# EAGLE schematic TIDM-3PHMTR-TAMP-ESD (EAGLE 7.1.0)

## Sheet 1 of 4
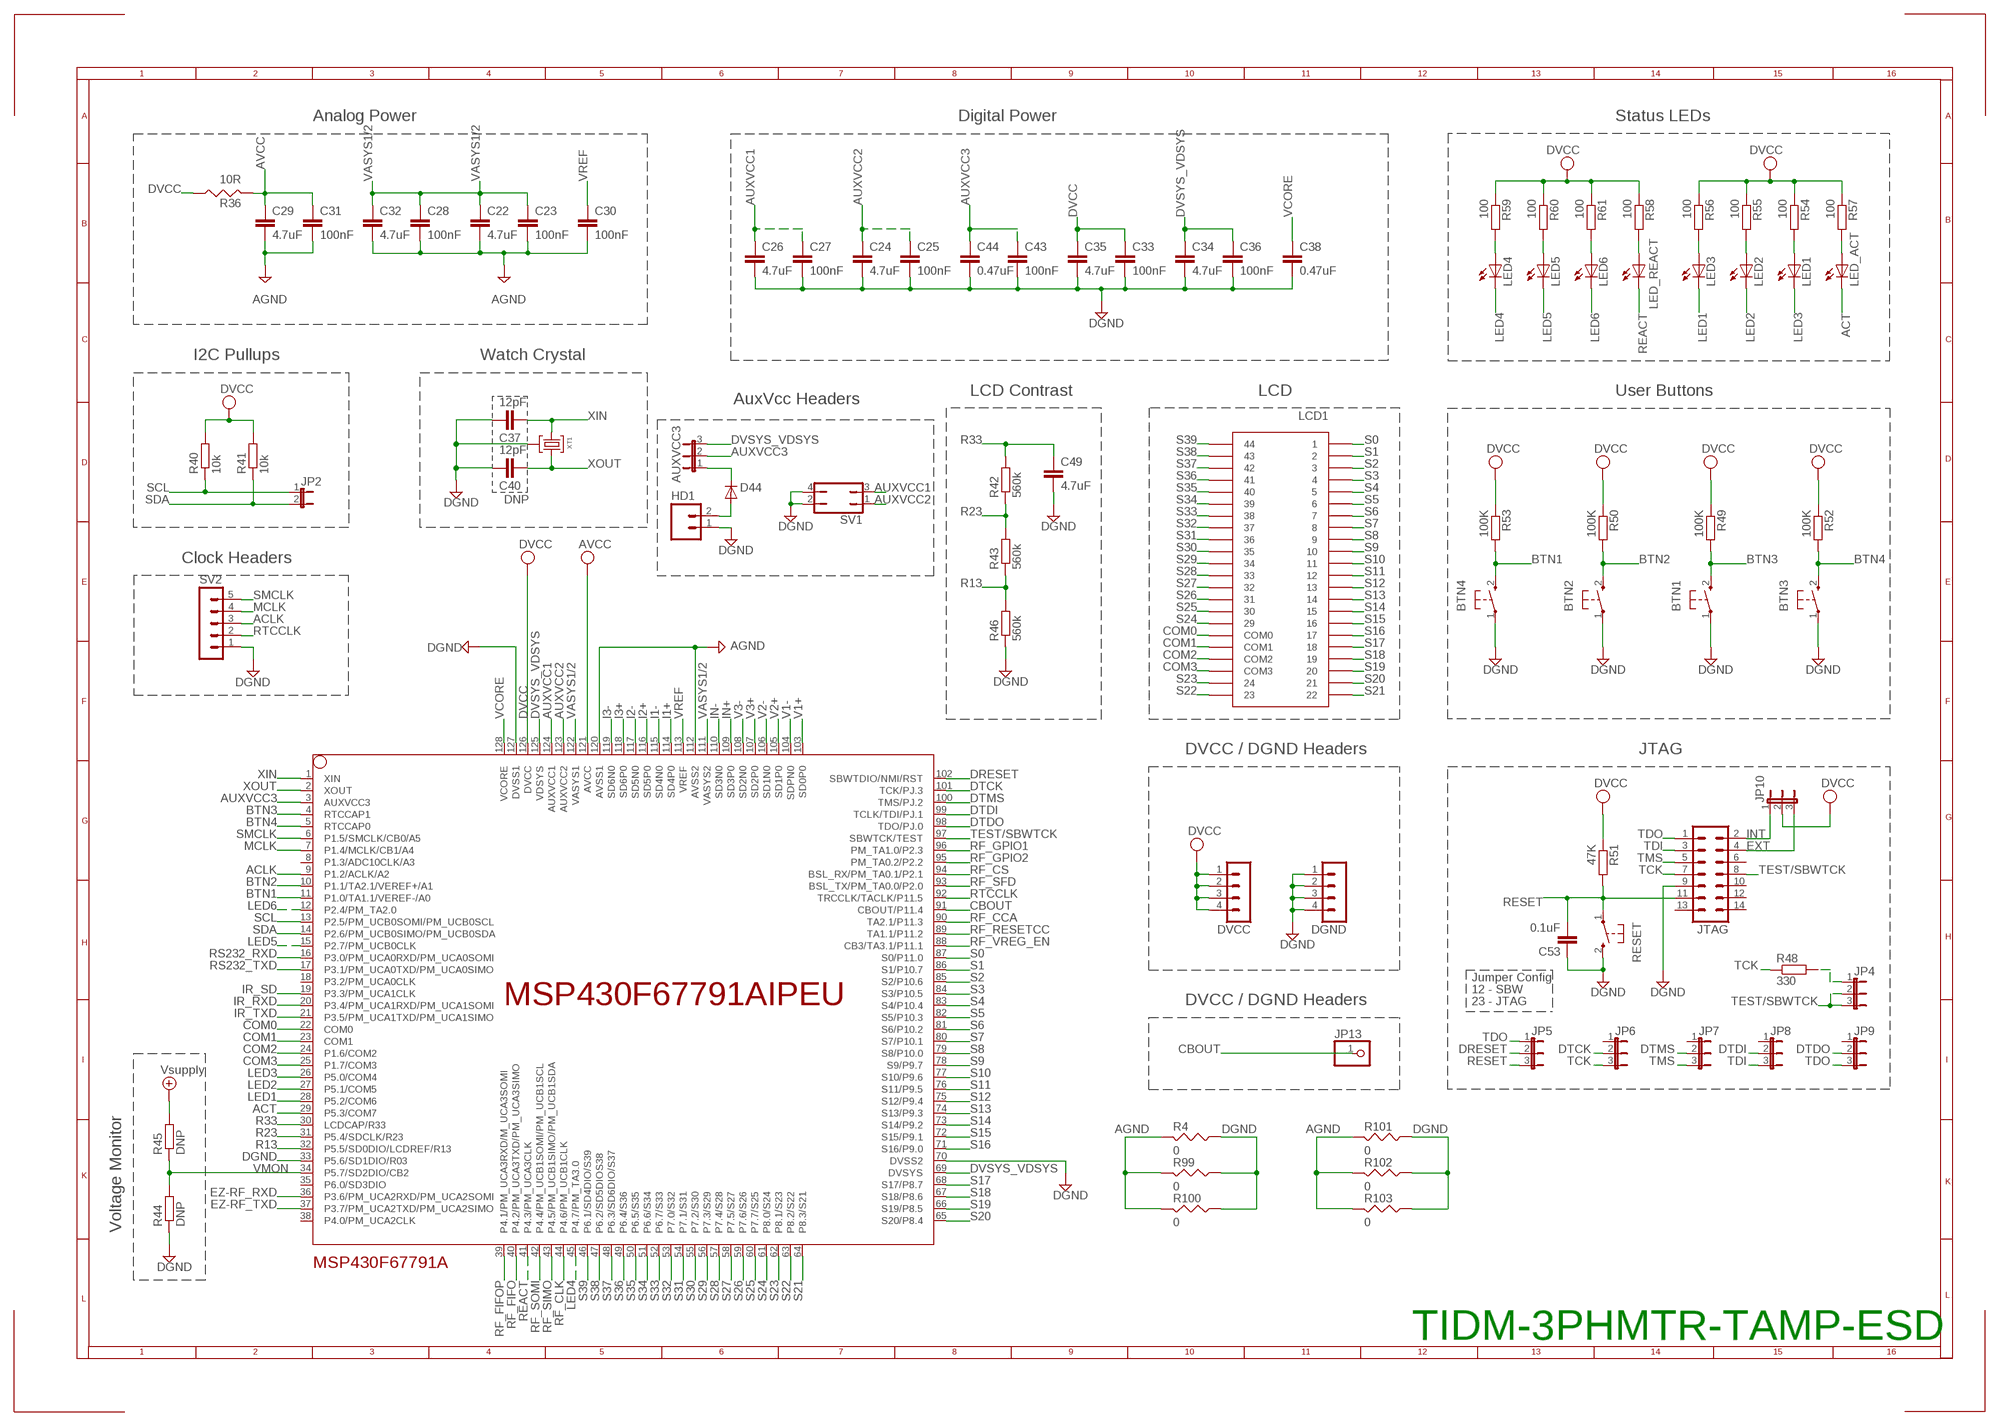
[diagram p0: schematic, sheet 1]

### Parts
AUXVCC3  JP2E  [JP2]
BTN1  PB  [PBTH]
BTN2  PB  [PBTH]
BTN3  PB  [PBTH]
BTN4  PB  [PBTH]
C22  4.7uF  C-EUC0603  [C0603]
C23  100nF  C-EUC0603  [C0603]
C24  4.7uF  C-EUC0603  [C0603]
C25  100nF  C-EUC0603  [C0603]
C26  4.7uF  C-EUC0603  [C0603]
C27  100nF  C-EUC0603  [C0603]
C28  100nF  C-EUC0603  [C0603]
C29  4.7uF  C-EUC0603  [C0603]
C30  100nF  C-EUC0603  [C0603]
C31  100nF  C-EUC0603  [C0603]
C32  4.7uF  C-EUC0603  [C0603]
C33  100nF  C-EUC0603  [C0603]
C34  4.7uF  C-EUC0603  [C0603]
C35  4.7uF  C-EUC0603  [C0603]
C36  100nF  C-EUC0603  [C0603]
C37  12pF  C-EUC0603  [C0603]
C38  0.47uF  C-EUC0603  [C0603]
C40  12pF  C-EUC0603  [C0603]
C43  100nF  C-EUC0603  [C0603]
C44  0.47uF  C-EUC0603  [C0603]
C49  4.7uF  C-EUC0603  [C0603]
C53  0.1uF  C-EUC0603  [C0603]
D44  PMLL4148  [SOD80C]
DGND  MA04-1  [MA04-1]
DVCC  MA04-1  [MA04-1]
HD1  M02PTH  [1X02]
JP2  JP1E  [JP1]
JP4  JP2E  [JP2]
JP5  JP2E  [JP2]
JP6  JP2E  [JP2]
JP7  JP2E  [JP2]
JP8  JP2E  [JP2]
JP9  JP2E  [JP2]
JP10  JP2E  [JP2]
JP13  PINHD-1X1  [1X01]
JTAG  ML14  [ML14]
LCD1  TI_160SEG_LCD  [TI_160SEG_LCD]
LED1  LED3MM  [LED3MM]
LED2  LED3MM  [LED3MM]
LED3  LED3MM  [LED3MM]
LED4  LED3MM  [LED3MM]
LED5  LED3MM  [LED3MM]
LED6  LED3MM  [LED3MM]
LED_ACT  LED3MM  [LED3MM]
LED_REACT  LED3MM  [LED3MM]
MSP430F67791A  MSP430F6779IPEU  [PEU128]
R4  0  RES0805  [R0805]
R36  10R  RES0805  [R0805]
R40  10k  R-EU_R0603  [R0603]
R41  10k  R-EU_R0603  [R0603]
R42  560k  R-EU_R0603  [R0603]
R43  560k  R-EU_R0603  [R0603]
R44  DNP  R-EU_R0603  [R0603]
R45  DNP  R-EU_R0603  [R0603]
R46  560k  R-EU_R0603  [R0603]
R48  330  R-EU_R0603  [R0603]
R49  100K  R-EU_R0603  [R0603]
R50  100K  R-EU_R0603  [R0603]
R51  47K  R-EU_R0603  [R0603]
R52  100K  R-EU_R0603  [R0603]
R53  100K  R-EU_R0603  [R0603]
R54  100  R-EU_R0603  [R0603]
R55  100  R-EU_R0603  [R0603]
R56  100  R-EU_R0603  [R0603]
R57  100  R-EU_R0603  [R0603]
R58  100  R-EU_R0603  [R0603]
R59  100  R-EU_R0603  [R0603]
R60  100  R-EU_R0603  [R0603]
R61  100  R-EU_R0603  [R0603]
R99  0  RES0805  [R0805]
R100  0  RES0805  [R0805]
R101  0  RES0805  [R0805]
R102  0  RES0805  [R0805]
R103  0  RES0805  [R0805]
RESET  PB  [PBTH]
SV1  JP2Q  [JP2Q]
SV2  MA05-1  [MA05-1]
XT1  CM200T  [CM200T]

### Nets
ACLK: MSP430F67791A.9(P1.2/ACLK/A2) SV2.3
ACT: LED_ACT.K(C) MSP430F67791A.29(P5.3/COM7) ; also sheet 4
AGND: C22.2 C23.2 C28.2 C29.2 C30.2 C31.2 C32.2 MSP430F67791A.112(AVSS2) MSP430F67791A.120(AVSS1) R4.2 R99.2 R100.2 R101.2 R102.2 R103.2 ; also sheet 2
AUXVCC1: C26.1 C27.1 MSP430F67791A.124(AUXVCC1) SV1.3
AUXVCC2: C24.1 C25.1 MSP430F67791A.123(AUXVCC2) SV1.1
AUXVCC3: AUXVCC3.2 C43.1 C44.1 MSP430F67791A.3(AUXVCC3)
AVCC: C29.1 C31.1 MSP430F67791A.121(AVCC) R36.2 ; also sheet 2
BTN1: BTN4.2(S) MSP430F67791A.11(P1.0/TA1.1/VEREF-/A0) R53.2
BTN2: BTN2.2(S) MSP430F67791A.10(P1.1/TA2.1/VEREF+/A1) R50.2
BTN3: BTN1.2(S) MSP430F67791A.4(RTCCAP1) R49.2
BTN4: BTN3.2(S) MSP430F67791A.5(RTCCAP0) R52.2
CBOUT: JP13.1 MSP430F67791A.91(CBOUT/P11.4)
COM0: LCD1.COM0 MSP430F67791A.22(COM0)
COM1: LCD1.COM1 MSP430F67791A.23(COM1)
COM2: LCD1.COM2 MSP430F67791A.24(P1.6/COM2)
COM3: LCD1.COM3 MSP430F67791A.25(P1.7/COM3)
DGND: BTN1.1(P) BTN2.1(P) BTN3.1(P) BTN4.1(P) C24.2 C25.2 C26.2 C27.2 C33.2 C34.2 C35.2 C36.2 C37.2 C38.2 C40.2 C43.2 C44.2 C49.2 C53.1 DGND.1 DGND.2 DGND.3 DGND.4 HD1.1 JTAG.9 MSP430F67791A.33(P5.6/SD1DIO/R03) MSP430F67791A.70(DVSS2) MSP430F67791A.127(DVSS1) R4.1 R44.1 R46.1 R99.1 R100.1 R101.1 R102.1 R103.1 RESET.2(S) SV1.2 SV1.4 SV2.1 XT1.P3 ; also sheet 3,4
DRESET: JP5.2 MSP430F67791A.102(SBWTDIO/NMI/RST)
DTCK: JP6.2 MSP430F67791A.101(TCK/PJ.3)
DTDI: JP8.2 MSP430F67791A.99(TCLK/TDI/PJ.1)
DTDO: JP9.2 MSP430F67791A.98(TDO/PJ.0)
DTMS: JP7.2 MSP430F67791A.100(TMS/PJ.2)
DVCC: C33.1 C35.1 DVCC.1 DVCC.2 DVCC.3 DVCC.4 JP10.2 MSP430F67791A.126(DVCC) R36.1 R40.2 R41.2 R49.1 R50.1 R51.1 R52.1 R53.1 R54.1 R55.1 R56.1 R57.1 R58.1 R59.1 R60.1 R61.1 ; also sheet 3,4
DVSYS_VDSYS: AUXVCC3.3 C34.1 C36.1 MSP430F67791A.69(DVSYS) MSP430F67791A.125(VDSYS)
EXT: JP10.3 JTAG.4
EZ-RF_RXD: MSP430F67791A.36(P3.6/PM_UCA2RXD/PM_UCA2SOMI) ; also sheet 4
EZ-RF_TXD: MSP430F67791A.37(P3.7/PM_UCA2TXD/PM_UCA2SIMO) ; also sheet 4
I1+: MSP430F67791A.114(SD4P0) ; also sheet 2
I1-: MSP430F67791A.115(SD4N0) ; also sheet 2
I2+: MSP430F67791A.116(SD5P0) ; also sheet 2
I2-: MSP430F67791A.117(SD5N0) ; also sheet 2
I3+: MSP430F67791A.118(SD6P0) ; also sheet 2
I3-: MSP430F67791A.119(SD6N0) ; also sheet 2
IN+: MSP430F67791A.109(SD3P0) ; also sheet 2
IN-: MSP430F67791A.110(SD3N0) ; also sheet 2
INT: JP10.1 JTAG.2
IR_RXD: MSP430F67791A.20(P3.4/PM_UCA1RXD/PM_UCA1SOMI) ; also sheet 4
IR_SD: MSP430F67791A.19(P3.3/PM_UCA1CLK) ; also sheet 4
IR_TXD: MSP430F67791A.21(P3.5/PM_UCA1TXD/PM_UCA1SIMO) ; also sheet 4
LED1: LED3.K(C) MSP430F67791A.28(P5.2/COM6)
LED2: LED2.K(C) MSP430F67791A.27(P5.1/COM5)
LED3: LED1.K(C) MSP430F67791A.26(P5.0/COM4)
LED4: LED4.K(C) MSP430F67791A.45(P4.7/PM_TA3.0)
LED5: LED5.K(C) MSP430F67791A.15(P2.7/PM_UCB0CLK)
LED6: LED6.K(C) MSP430F67791A.12(P2.4/PM_TA2.0)
MCLK: MSP430F67791A.7(P1.4/MCLK/CB1/A4) SV2.4
N$4: LED3.A R56.2
N$5: AUXVCC3.1 D44.C
N$7: LED2.A R55.2
N$10: JP4.1 R48.2
N$21: LED4.A R59.2
N$27: LED5.A R60.2
N$30: LED1.A R54.2
N$36: LED6.A R61.2
N$44: LED_REACT.A R58.2
N$46: LED_ACT.A R57.2
N$49: D44.A HD1.2
R13: MSP430F67791A.32(P5.5/SD0DIO/LCDREF/R13) R43.1 R46.2
R23: MSP430F67791A.31(P5.4/SDCLK/R23) R42.1 R43.2
R33: C49.1 MSP430F67791A.30(LCDCAP/R33) R42.2
REACT: LED_REACT.K(C) MSP430F67791A.41(P4.3/PM_UCA3CLK) ; also sheet 4
RESET: C53.2 JP5.3 JTAG.11 R51.2 RESET.1(P)
RF_CCA: MSP430F67791A.90(TA2.1/P11.3) ; also sheet 4
RF_CLK: MSP430F67791A.44(P4.6/PM_UCB1CLK) ; also sheet 4
RF_CS: MSP430F67791A.94(BSL_RX/PM_TA0.1/P2.1) ; also sheet 4
RF_FIFO: MSP430F67791A.40(P4.2/PM_UCA3TXD/PM_UCA3SIMO) ; also sheet 4
RF_FIFOP: MSP430F67791A.39(P4.1/PM_UCA3RXD/M_UCA3SOMI) ; also sheet 4
RF_GPIO1: MSP430F67791A.96(PM_TA1.0/P2.3) ; also sheet 4
RF_GPIO2: MSP430F67791A.95(PM_TA0.2/P2.2) ; also sheet 4
RF_RESETCC: MSP430F67791A.89(TA1.1/P11.2) ; also sheet 4
RF_SFD: MSP430F67791A.93(BSL_TX/PM_TA0.0/P2.0) ; also sheet 4
RF_SIMO: MSP430F67791A.43(P4.5/PM_UCB1SIMO/PM_UCB1SDA) ; also sheet 4
RF_SOMI: MSP430F67791A.42(P4.4/PM_UCB1SOMI/PM_UCB1SCL) ; also sheet 4
RF_VREG_EN: MSP430F67791A.88(CB3/TA3.1/P11.1) ; also sheet 4
RS232_RXD: MSP430F67791A.16(P3.0/PM_UCA0RXD/PM_UCA0SOMI) ; also sheet 4
RS232_TXD: MSP430F67791A.17(P3.1/PM_UCA0TXD/PM_UCA0SIMO) ; also sheet 4
RTCCLK: MSP430F67791A.92(TRCCLK/TACLK/P11.5) SV2.2
S0: LCD1.1 MSP430F67791A.87(S0/P11.0)
S1: LCD1.2 MSP430F67791A.86(S1/P10.7)
S2: LCD1.3 MSP430F67791A.85(S2/P10.6)
S3: LCD1.4 MSP430F67791A.84(S3/P10.5)
S4: LCD1.5 MSP430F67791A.83(S4/P10.4)
S5: LCD1.6 MSP430F67791A.82(S5/P10.3)
S6: LCD1.7 MSP430F67791A.81(S6/P10.2)
S7: LCD1.8 MSP430F67791A.80(S7/P10.1)
S8: LCD1.9 MSP430F67791A.79(S8/P10.0)
S9: LCD1.10 MSP430F67791A.78(S9/P9.7)
S10: LCD1.11 MSP430F67791A.77(S10/P9.6)
S11: LCD1.12 MSP430F67791A.76(S11/P9.5)
S12: LCD1.13 MSP430F67791A.75(S12/P9.4)
S13: LCD1.14 MSP430F67791A.74(S13/P9.3)
S14: LCD1.15 MSP430F67791A.73(S14/P9.2)
S15: LCD1.16 MSP430F67791A.72(S15/P9.1)
S16: LCD1.17 MSP430F67791A.71(S16/P9.0)
S17: LCD1.18 MSP430F67791A.68(S17/P8.7)
S18: LCD1.19 MSP430F67791A.67(S18/P8.6)
S19: LCD1.20 MSP430F67791A.66(S19/P8.5)
S20: LCD1.21 MSP430F67791A.65(S20/P8.4)
S21: LCD1.22 MSP430F67791A.64(P8.3/S21)
S22: LCD1.23 MSP430F67791A.63(P8.2/S22)
S23: LCD1.24 MSP430F67791A.62(P8.1/S23)
S24: LCD1.29 MSP430F67791A.61(P8.0/S24)
S25: LCD1.30 MSP430F67791A.60(P7.7/S25)
S26: LCD1.31 MSP430F67791A.59(P7.6/S26)
S27: LCD1.32 MSP430F67791A.58(P7.5/S27)
S28: LCD1.33 MSP430F67791A.57(P7.4/S28)
S29: LCD1.34 MSP430F67791A.56(P7.3/S29)
S30: LCD1.35 MSP430F67791A.55(P7.2/S30)
S31: LCD1.36 MSP430F67791A.54(P7.1/S31)
S32: LCD1.37 MSP430F67791A.53(P7.0/S32)
S33: LCD1.38 MSP430F67791A.52(P6.7/S33)
S34: LCD1.39 MSP430F67791A.51(P6.6/S34)
S35: LCD1.40 MSP430F67791A.50(P6.5/S35)
S36: LCD1.41 MSP430F67791A.49(P6.4/S36)
S37: LCD1.42 MSP430F67791A.48(P6.3/SD6DIO/S37)
S38: LCD1.43 MSP430F67791A.47(P6.2/SD5DIOS38)
S39: LCD1.44 MSP430F67791A.46(P6.1/SD4DIO/S39)
SCL: JP2.1 MSP430F67791A.13(P2.5/PM_UCB0SOMI/PM_UCB0SCL) R40.1 ; also sheet 4
SDA: JP2.2 MSP430F67791A.14(P2.6/PM_UCB0SIMO/PM_UCB0SDA) R41.1 ; also sheet 4
SMCLK: MSP430F67791A.6(P1.5/SMCLK/CB0/A5) SV2.5
TCK: JP6.3 JTAG.7 R48.1
TDI: JP8.3 JTAG.3
TDO: JP5.1 JP9.3 JTAG.1
TEST/SBWTCK: JP4.2 JP4.3 JTAG.8 MSP430F67791A.97(SBWTCK/TEST)
TMS: JP7.3 JTAG.5
V1+: MSP430F67791A.103(SD0P0) ; also sheet 2
V1-: MSP430F67791A.104(SDPN0) ; also sheet 2
V2+: MSP430F67791A.105(SD1P0) ; also sheet 2
V2-: MSP430F67791A.106(SD1N0) ; also sheet 2
V3+: MSP430F67791A.107(SD2P0) ; also sheet 2
V3-: MSP430F67791A.108(SD2N0) ; also sheet 2
VASYS1/2: C22.1 C23.1 C28.1 C32.1 MSP430F67791A.111(VASYS2) MSP430F67791A.122(VASYS1)
VCORE: C38.1 MSP430F67791A.128(VCORE)
VMON: MSP430F67791A.34(P5.7/SD2DIO/CB2) R44.2 R45.1
VREF: C30.1 MSP430F67791A.113(VREF)
VSUPPLY: R45.2 ; supply symbol labelled Vsupply ; also sheet 3
XIN: C37.1 MSP430F67791A.1(XIN) XT1.P2
XOUT: C40.1 MSP430F67791A.2(XOUT) XT1.P1
Unconnected: JP6.1 JP7.1 JP8.1 JP9.1 JTAG.6 JTAG.10 JTAG.12 JTAG.13 JTAG.14 MSP430F67791A.8(P1.3/ADC10CLK/A3) MSP430F67791A.18(P3.2/PM_UCA0CLK) MSP430F67791A.35(P6.0/SD3DIO) MSP430F67791A.38(P4.0/PM_UCA2CLK)

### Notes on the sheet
- Analog Power | Digital Power | Status LEDs
- I2C Pullups | Watch Crystal
- LCD Contrast | LCD | User Buttons
- AuxVcc Headers
- DNP
- Clock Headers
- DVCC / DGND Headers | JTAG
- Jumper Config
- 12 - SBW
- DVCC / DGND Headers | 23 - JTAG
- Voltage Monitor
- TIDM-3PHMTR-TAMP-ESD

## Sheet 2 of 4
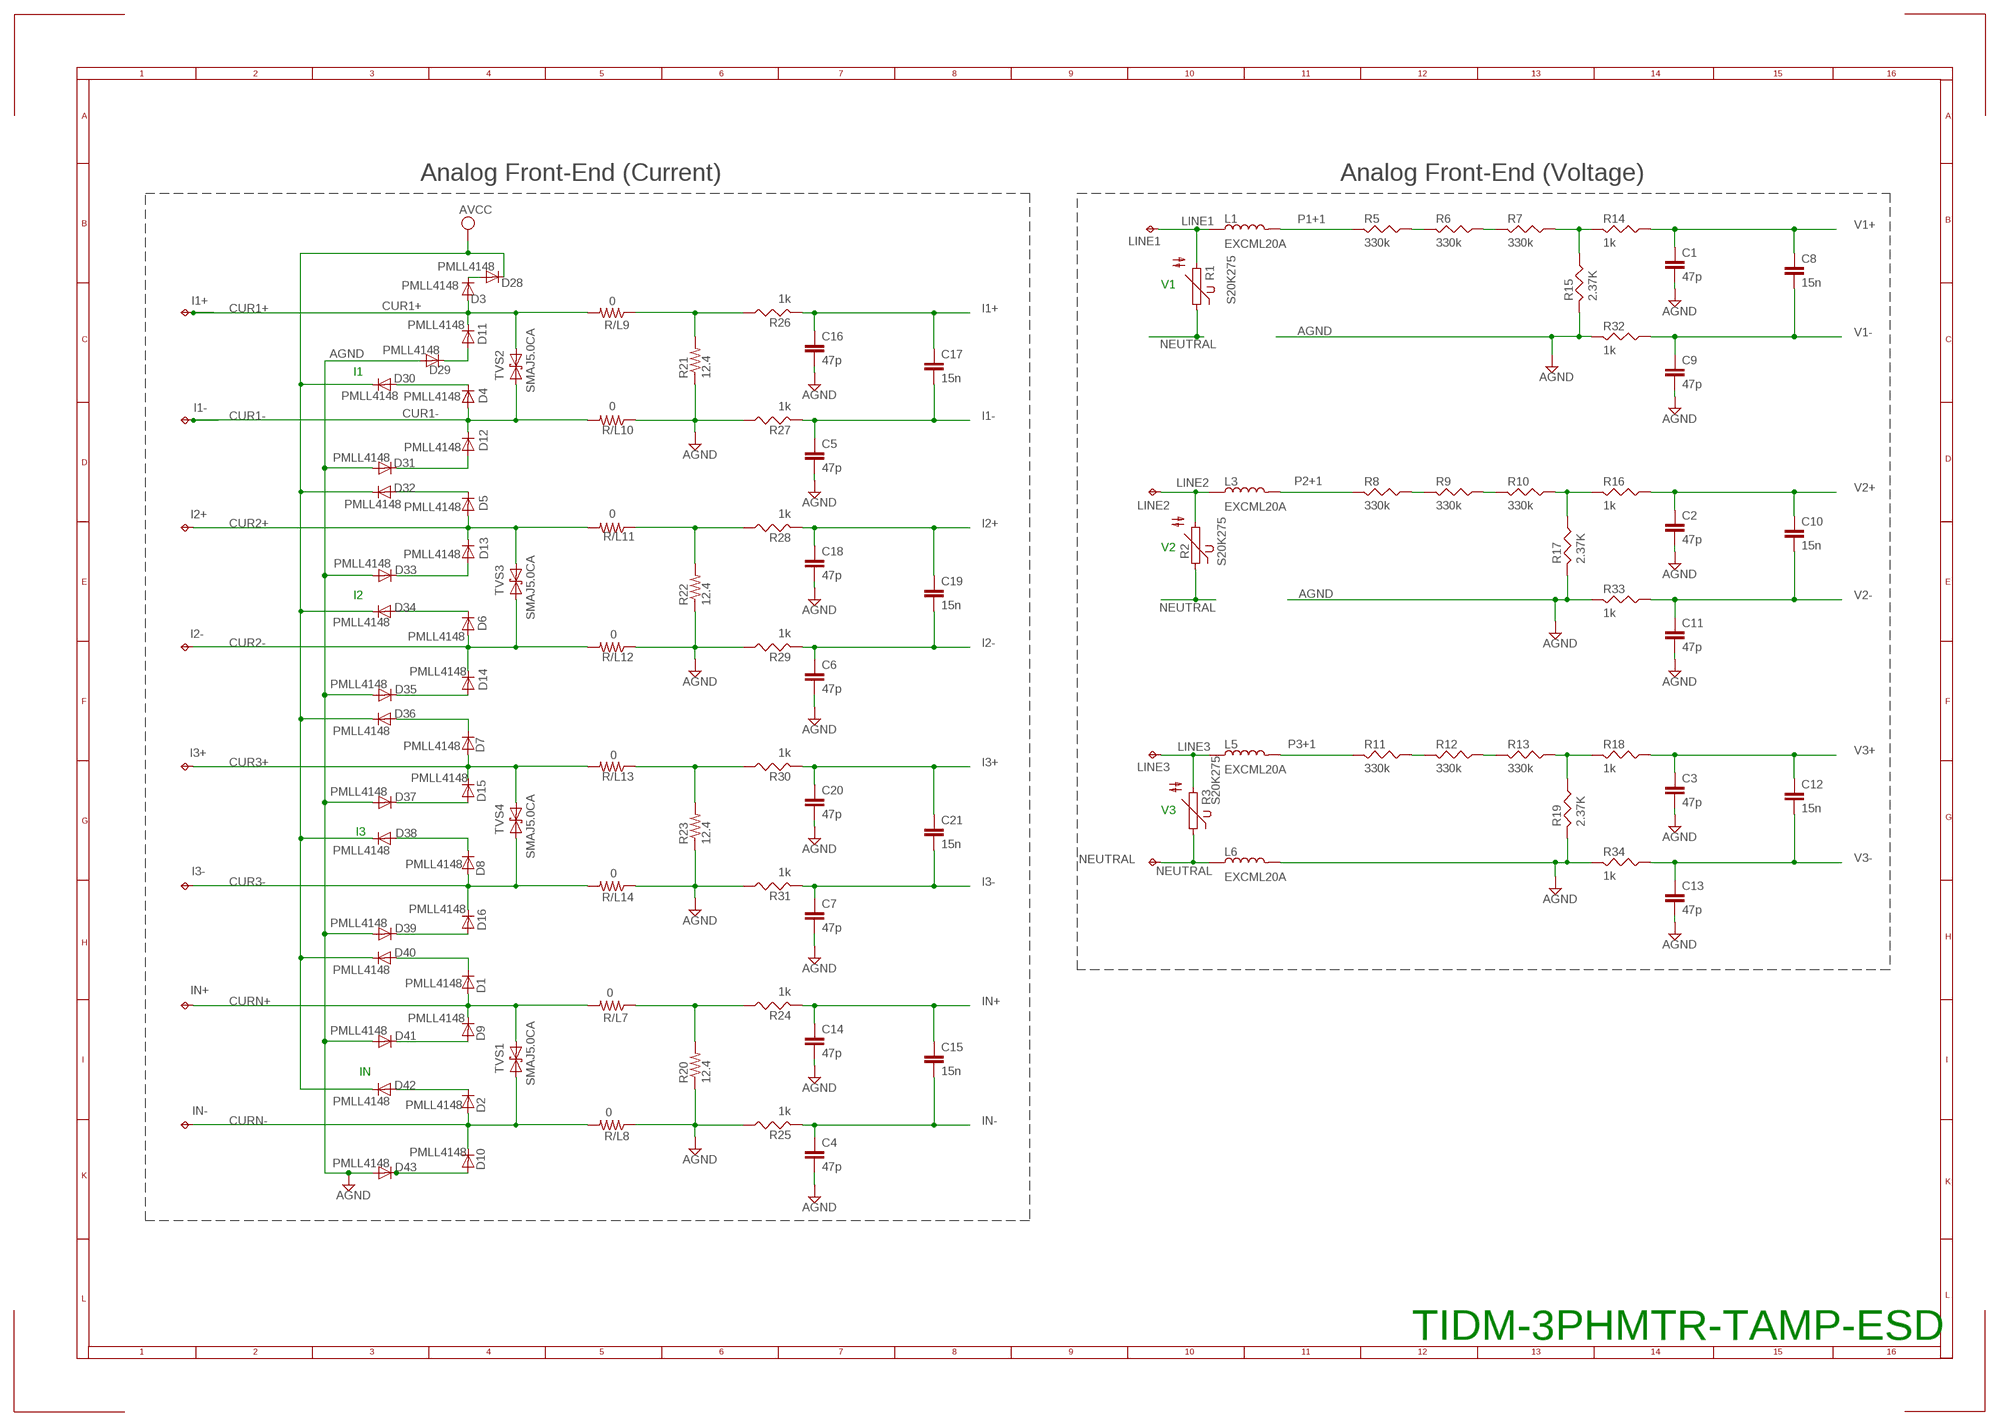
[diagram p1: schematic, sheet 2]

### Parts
C1  47p  C-EUC0805  [C0805]
C2  47p  C-EUC0805  [C0805]
C3  47p  C-EUC0805  [C0805]
C4  47p  C-EUC0805  [C0805]
C5  47p  C-EUC0805  [C0805]
C6  47p  C-EUC0805  [C0805]
C7  47p  C-EUC0805  [C0805]
C8  15n  C-EUC0805  [C0805]
C9  47p  C-EUC0805  [C0805]
C10  15n  C-EUC0805  [C0805]
C11  47p  C-EUC0805  [C0805]
C12  15n  C-EUC0805  [C0805]
C13  47p  C-EUC0805  [C0805]
C14  47p  C-EUC0805  [C0805]
C15  15n  C-EUC0805  [C0805]
C16  47p  C-EUC0805  [C0805]
C17  15n  C-EUC0805  [C0805]
C18  47p  C-EUC0805  [C0805]
C19  15n  C-EUC0805  [C0805]
C20  47p  C-EUC0805  [C0805]
C21  15n  C-EUC0805  [C0805]
D1  PMLL4148  [SOD80C]
D2  PMLL4148  [SOD80C]
D3  PMLL4148  [SOD80C]
D4  PMLL4148  [SOD80C]
D5  PMLL4148  [SOD80C]
D6  PMLL4148  [SOD80C]
D7  PMLL4148  [SOD80C]
D8  PMLL4148  [SOD80C]
D9  PMLL4148  [SOD80C]
D10  PMLL4148  [SOD80C]
D11  PMLL4148  [SOD80C]
D12  PMLL4148  [SOD80C]
D13  PMLL4148  [SOD80C]
D14  PMLL4148  [SOD80C]
D15  PMLL4148  [SOD80C]
D16  PMLL4148  [SOD80C]
D28  PMLL4148  [SOD80C]
D29  PMLL4148  [SOD80C]
D30  PMLL4148  [SOD80C]
D31  PMLL4148  [SOD80C]
D32  PMLL4148  [SOD80C]
D33  PMLL4148  [SOD80C]
D34  PMLL4148  [SOD80C]
D35  PMLL4148  [SOD80C]
D36  PMLL4148  [SOD80C]
D37  PMLL4148  [SOD80C]
D38  PMLL4148  [SOD80C]
D39  PMLL4148  [SOD80C]
D40  PMLL4148  [SOD80C]
D41  PMLL4148  [SOD80C]
D42  PMLL4148  [SOD80C]
D43  PMLL4148  [SOD80C]
I1+  TPPAD1-20  [P1-20]
I1-  TPPAD1-20  [P1-20]
I2+  TPPAD1-20  [P1-20]
I2-  TPPAD1-20  [P1-20]
I3+  TPPAD1-20  [P1-20]
I3-  TPPAD1-20  [P1-20]
IN+  TPPAD1-20  [P1-20]
IN-  TPPAD1-20  [P1-20]
L1  EXCML20A  EXCELSA390805  [R0805]
L3  EXCML20A  EXCELSA390805  [R0805]
L5  EXCML20A  EXCELSA390805  [R0805]
L6  EXCML20A  EXCELSA390805  [R0805]
LINE1  TPPAD1-20  [P1-20]
LINE2  TPPAD1-20  [P1-20]
LINE3  TPPAD1-20  [P1-20]
NEUTRAL  TPPAD1-20  [P1-20]
R1  S20K275  [S20K275]
R2  S20K275  [S20K275]
R3  S20K275  [S20K275]
R5  330k  RES0805  [R0805]
R6  330k  RES0805  [R0805]
R7  330k  RES0805  [R0805]
R8  330k  RES0805  [R0805]
R9  330k  RES0805  [R0805]
R10  330k  RES0805  [R0805]
R11  330k  RES0805  [R0805]
R12  330k  RES0805  [R0805]
R13  330k  RES0805  [R0805]
R14  1k  RES0805  [R0805]
R15  2.37K  RES0805  [R0805]
R16  1k  RES0805  [R0805]
R17  2.37K  RES0805  [R0805]
R18  1k  RES0805  [R0805]
R19  2.37K  RES0805  [R0805]
R20  12.4  R-US_R0805  [R0805]
R21  12.4  R-US_R0805  [R0805]
R22  12.4  R-US_R0805  [R0805]
R23  12.4  R-US_R0805  [R0805]
R24  1k  RES0805  [R0805]
R25  1k  RES0805  [R0805]
R26  1k  RES0805  [R0805]
R27  1k  RES0805  [R0805]
R28  1k  RES0805  [R0805]
R29  1k  RES0805  [R0805]
R30  1k  RES0805  [R0805]
R31  1k  RES0805  [R0805]
R32  1k  RES0805  [R0805]
R33  1k  RES0805  [R0805]
R34  1k  RES0805  [R0805]
R/L7  0  R-US_R0805  [R0805]
R/L8  0  R-US_R0805  [R0805]
R/L9  0  R-US_R0805  [R0805]
R/L10  0  R-US_R0805  [R0805]
R/L11  0  R-US_R0805  [R0805]
R/L12  0  R-US_R0805  [R0805]
R/L13  0  R-US_R0805  [R0805]
R/L14  0  R-US_R0805  [R0805]
TVS1  SMAJ5.0CA  [DO214AC]
TVS2  SMAJ5.0CA  [DO214AC]
TVS3  SMAJ5.0CA  [DO214AC]
TVS4  SMAJ5.0CA  [DO214AC]

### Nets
AGND: C1.2 C2.2 C3.2 C4.2 C5.2 C6.2 C7.2 C9.2 C11.2 C13.2 C14.2 C16.2 C18.2 C20.2 D29.A D31.A D33.A D35.A D37.A D39.A D41.A D43.A L6.2 R15.2 R17.2 R19.2 R20.1 R21.1 R22.1 R23.1 R25.1 R27.1 R29.1 R31.1 R32.2 R33.2 R34.2 R/L8.1 R/L10.1 R/L12.1 R/L14.1 ; also sheet 1
AVCC: D28.C D30.C D32.C D34.C D36.C D38.C D40.C D42.C ; also sheet 1
CUR1+: D3.A D11.C I1+.TP R/L9.2 TVS2.C(K)
CUR1-: D4.A D12.C I1-.TP R/L10.2 TVS2.A
CUR2+: D5.A D13.C I2+.TP R/L11.2 TVS3.C(K)
CUR2-: D6.A D14.C I2-.TP R/L12.2 TVS3.A
CUR3+: D7.A D15.C I3+.TP R/L13.2 TVS4.C(K)
CUR3-: D8.A D16.C I3-.TP R/L14.2 TVS4.A
CURN+: D1.A D9.C IN+.TP R/L7.2 TVS1.C(K)
CURN-: D2.A D10.C IN-.TP R/L8.2 TVS1.A
I1+: C16.1 C17.1 R26.2 ; also sheet 1
I1-: C5.1 C17.2 R27.2 ; also sheet 1
I2+: C18.1 C19.1 R28.2 ; also sheet 1
I2-: C6.1 C19.2 R29.2 ; also sheet 1
I3+: C20.1 C21.1 R30.2 ; also sheet 1
I3-: C7.1 C21.2 R31.2 ; also sheet 1
IN+: C14.1 C15.1 R24.2 ; also sheet 1
IN-: C4.1 C15.2 R25.2 ; also sheet 1
LINE1: L1.1 LINE1.TP R1.2
LINE2: L3.1 LINE2.TP R2.2
LINE3: L5.1 LINE3.TP R3.2
N$6: R20.2 R24.1 R/L7.1
N$8: R5.1 R6.2
N$13: R6.1 R7.2
N$14: R7.1 R14.2 R15.1
N$15: R8.1 R9.2
N$16: R9.1 R10.2
N$19: R10.1 R16.2 R17.1
N$20: D3.C D28.A
N$23: D11.A D29.C
N$25: R23.2 R30.1 R/L13.1
N$29: R11.1 R12.2
N$31: R22.2 R28.1 R/L11.1
N$32: R21.2 R26.1 R/L9.1
N$33: R12.1 R13.2
N$34: R13.1 R18.2 R19.1
N$39: D4.C D30.A
N$40: D12.A D31.C
N$42: D5.C D32.A
N$54: D13.A D33.C
N$62: D6.C D34.A
N$63: D14.A D35.C
N$64: D7.C D36.A
N$66: D15.A D37.C
N$70: D8.C D38.A
N$73: D16.A D39.C
N$74: D1.C D40.A
N$75: D9.A D41.C
N$76: D2.C D42.A
N$77: D10.A D43.C
NEUTRAL: L6.1 NEUTRAL.TP R1.1 R2.1 R3.1 ; also sheet 3
P1+1: L1.2 R5.2 ; also sheet 3
P2+1: L3.2 R8.2 ; also sheet 3
P3+1: L5.2 R11.2 ; also sheet 3
V1+: C1.1 C8.1 R14.1 ; also sheet 1
V1-: C8.2 C9.1 R32.1 ; also sheet 1
V2+: C2.1 C10.1 R16.1 ; also sheet 1
V2-: C10.2 C11.1 R33.1 ; also sheet 1
V3+: C3.1 C12.1 R18.1 ; also sheet 1
V3-: C12.2 C13.1 R34.1 ; also sheet 1

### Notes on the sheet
- Analog Front-End (Current) | Analog Front-End (Voltage)
- V1
- I1
- V2
- I2
- V3
- I3
- IN
- TIDM-3PHMTR-TAMP-ESD

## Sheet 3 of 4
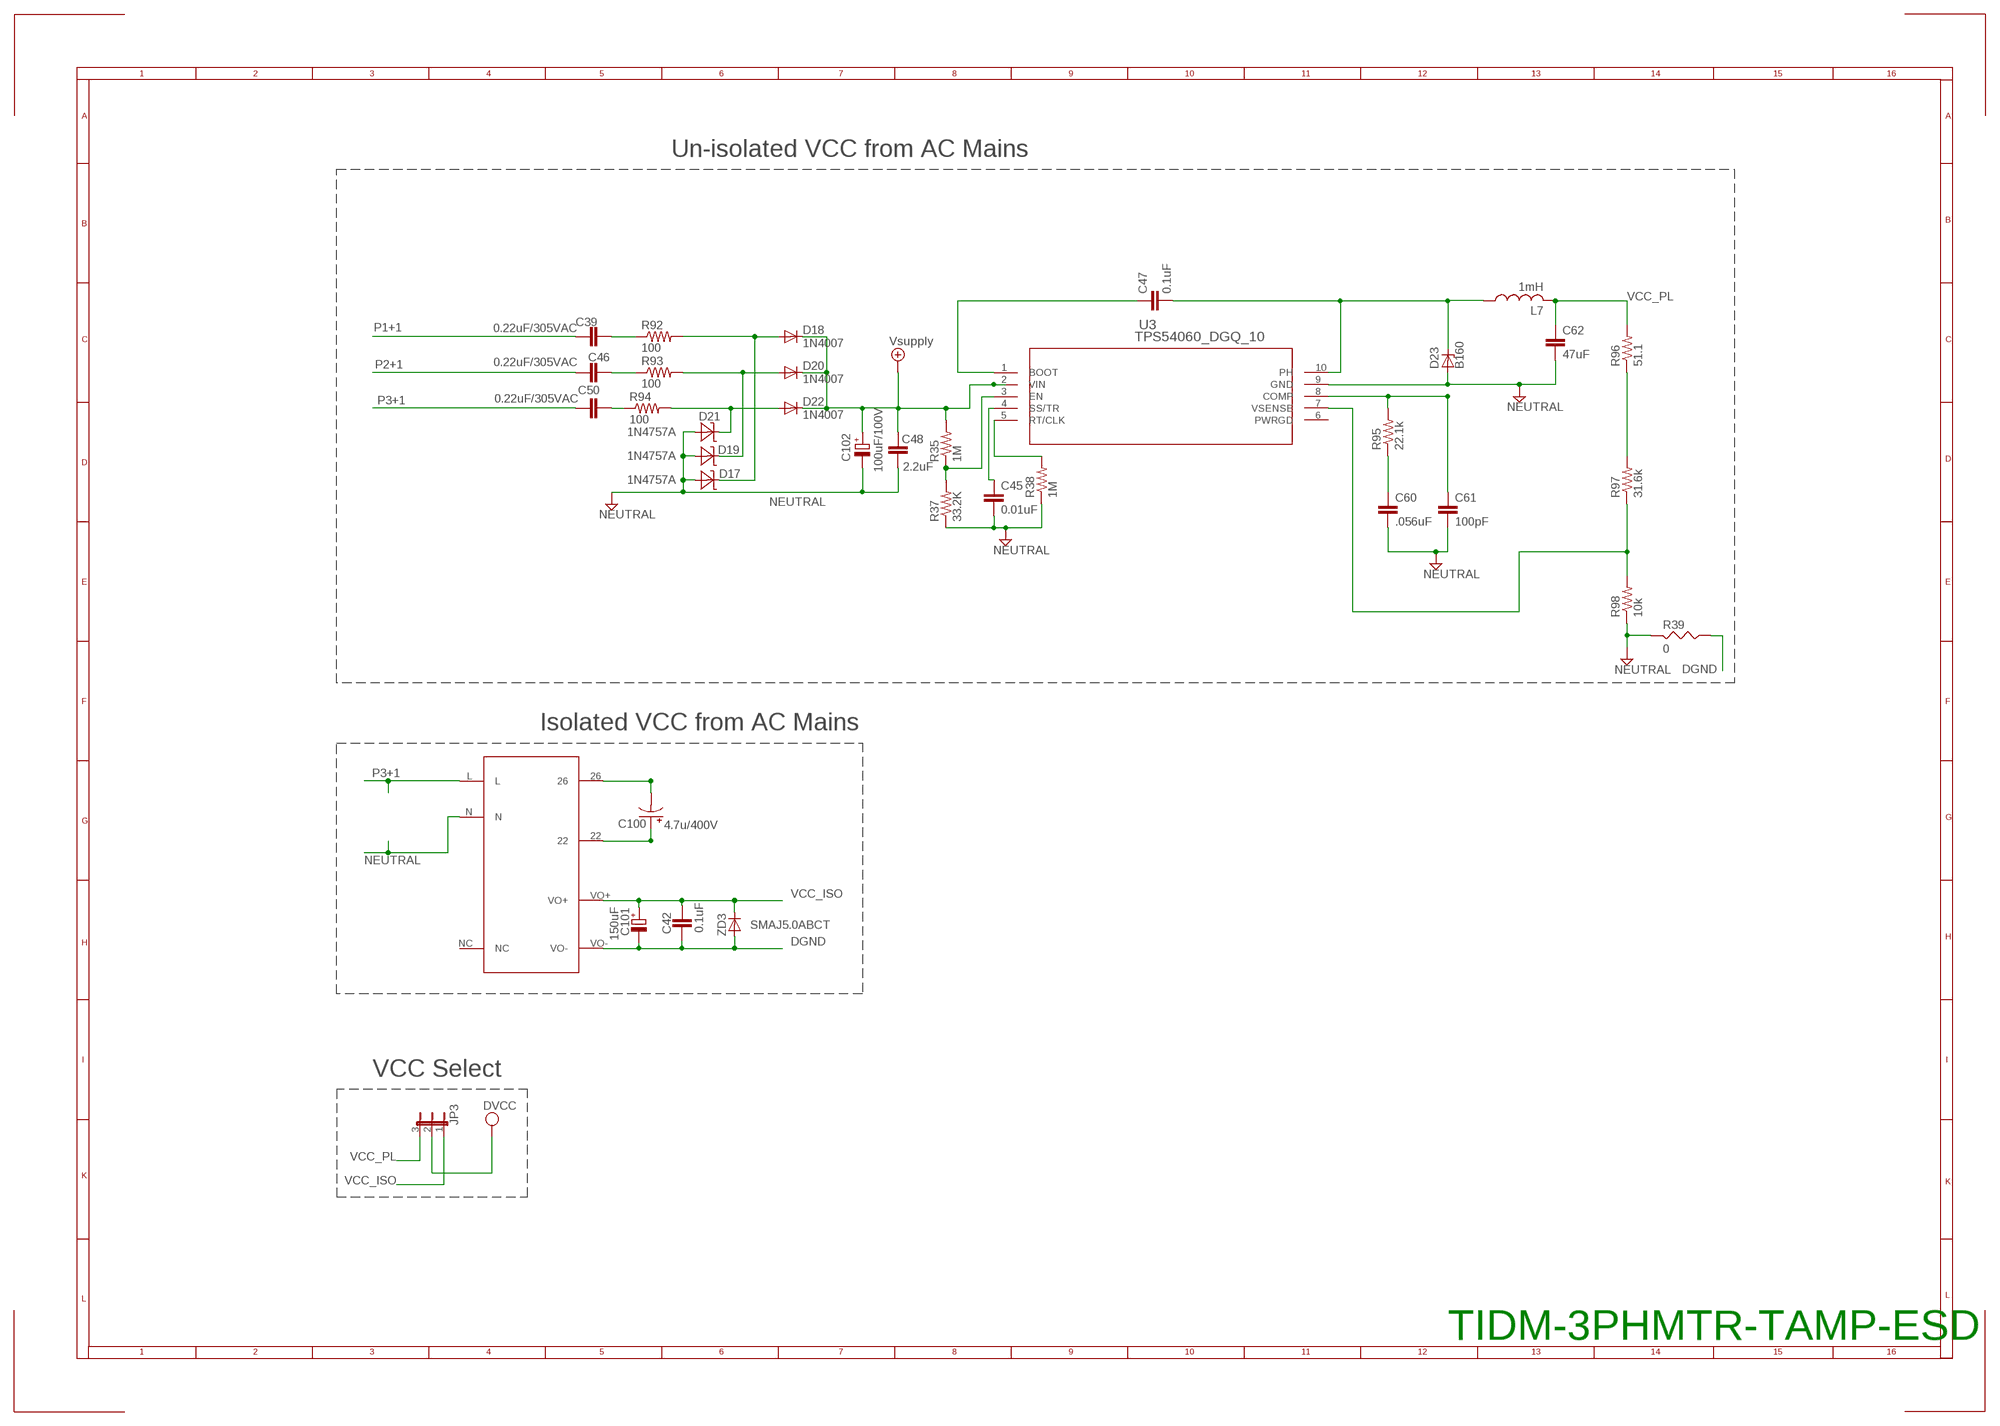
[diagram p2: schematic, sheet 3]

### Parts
C39  0.22uF/305VAC  C15/8  [C15B8]
C42  0.1uF  C-EUC0603  [C0603]
C45  0.01uF  C-EUC0603  [C0603]
C46  0.22uF/305VAC  C15/8  [C15B8]
C47  0.1uF  C-EUC0603  [C0603]
C48  2.2uF  C-EUC1210  [C1210]
C50  0.22uF/305VAC  C15/8  [C15B8]
C60  .056uF  C-EUC0603  [C0603]
C61  100pF  C-EUC0603  [C0603]
C62  47uF  C-EUC1210  [C1210]
C100  4.7u/400V  CPOL-USE5-10.5  [E5-10,5]
C101  150uF  CPOL-EUE2-5  [E2-5]
C102  100uF/100V  CPOL-EUE5-10.5  [E5-10,5]
D17  1N4757A  [DO41Z10]
D18  1N4007  [DO41-10]
D19  1N4757A  [DO41Z10]
D20  1N4007  [DO41-10]
D21  1N4757A  [DO41Z10]
D22  1N4007  [DO41-10]
D23  B160  ZENER-DIODESMB  [SMB]
JP3  JP2E  [JP2]
L7  1mH  L-USMSS1038-105  [INDUCTOR_POWER_SUPPLY_6779]
R35  1M  R-US_R0603  [R0603]
R37  33.2K  R-US_R0603  [R0603]
R38  1M  R-US_R0603  [R0603]
R39  0  RES0805  [R0805]
R92  100  R-US_0414/15  [0414/15]
R93  100  R-US_0414/15  [0414/15]
R94  100  R-US_0414/15  [0414/15]
R95  22.1k  R-US_R0603  [R0603]
R96  51.1  R-US_R0603  [R0603]
R97  31.6k  R-US_R0603  [R0603]
R98  10k  R-US_R0603  [R0603]
U3  TPS54060_DGQ_10  [DGQ10_1P88X1P57]
U$1  CUI_XR  [CUI_XR]
ZD3  SMAJ5.0ABCT  DIODE-DO214AC  [DO214AC]

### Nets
DGND: C42.2 C101.- R39.1 U$1.VO- ZD3.A ; also sheet 1,4
DVCC: JP3.2 ; also sheet 1,4
N$1: C100.- U$1.26
N$2: C100.+ U$1.22
N$17: R38.2 U3.5(RT/CLK)
N$18: D17.C D18.A R92.2
N$37: C45.1 U3.4(SS/TR)
N$38: R35.1 R37.2 U3.3(EN)
N$47: D19.C D20.A R93.2
N$78: C47.1 U3.1(BOOT)
N$80: C47.2 D23.C L7.1 U3.10(PH)
N$82: C60.1 R95.1
N$84: C39.2 R92.1
N$89: C46.2 R93.1
N$90: C50.2 R94.1
N$92: C61.1 R95.2 U3.8(COMP)
N$93: R96.1 R97.2
N$94: D21.C D22.A R94.2
N$95: R97.1 R98.2 U3.7(VSENSE)
NEUTRAL: C45.2 C48.2 C60.2 C61.2 C62.2 C102.- D17.A D19.A D21.A D23.A R37.1 R38.1 R39.2 R98.1 U3.9(GND) U$1.N ; also sheet 2
P1+1: C39.1 ; also sheet 2
P2+1: C46.1 ; also sheet 2
P3+1: C50.1 U$1.L ; also sheet 2
VCC_ISO: C42.1 C101.+ JP3.1 U$1.VO+ ZD3.C
VCC_PL: C62.1 JP3.3 L7.2 R96.2
VSUPPLY: C48.1 C102.+ D18.C D20.C D22.C R35.2 U3.2(VIN) ; supply symbol labelled Vsupply ; also sheet 1
Unconnected: U3.6(PWRGD) U$1.NC

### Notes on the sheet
- Un-isolated VCC from AC Mains
- Isolated VCC from AC Mains
- VCC Select
- TIDM-3PHMTR-TAMP-ESD

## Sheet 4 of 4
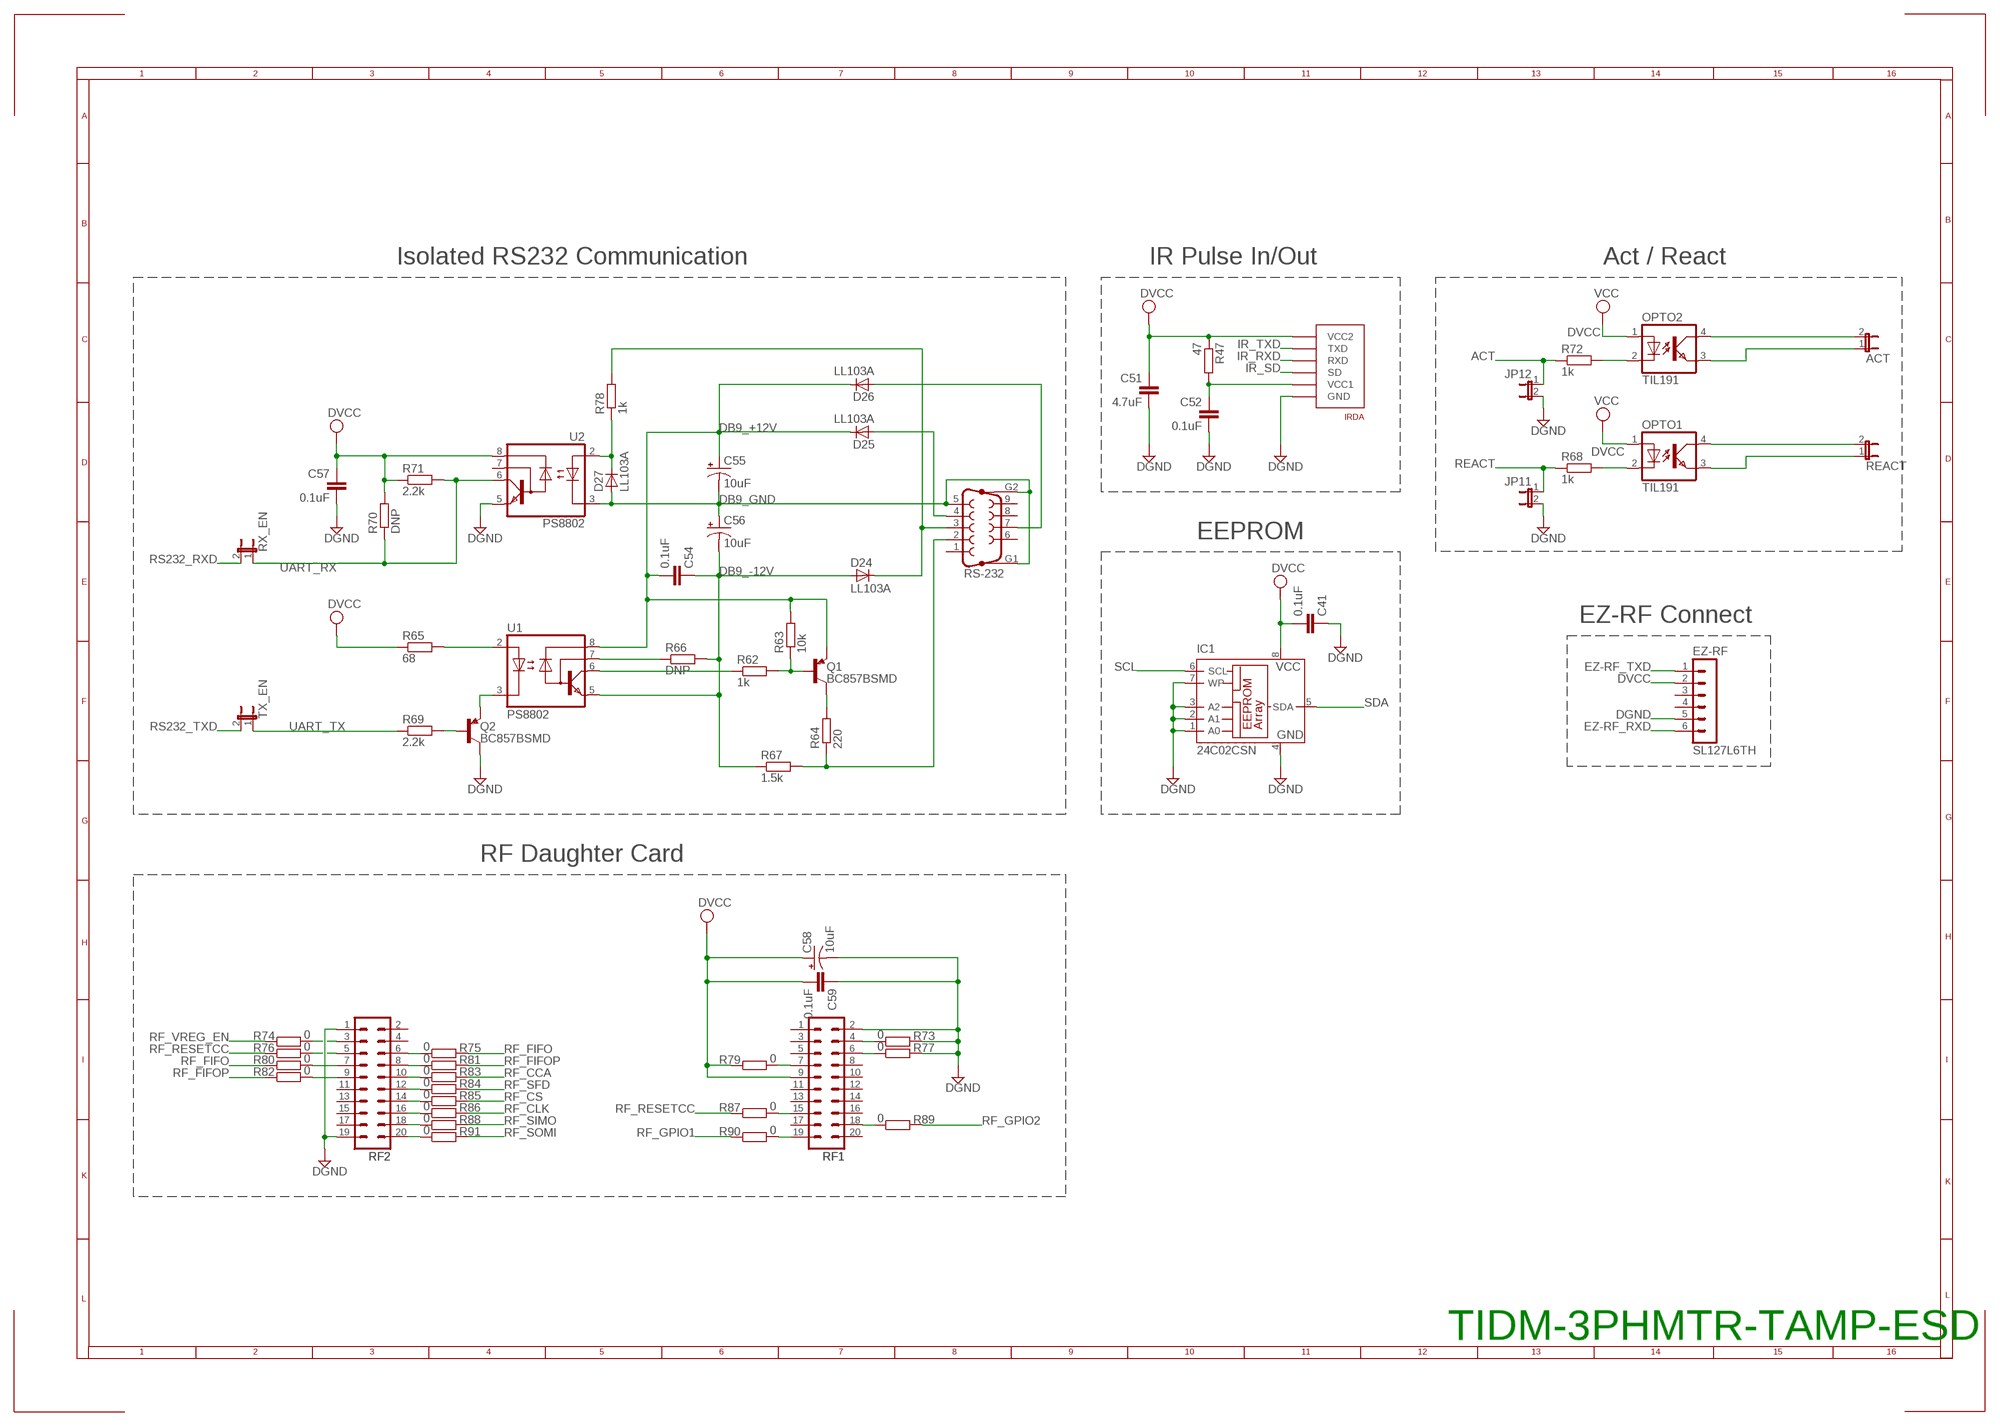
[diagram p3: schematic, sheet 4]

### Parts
ACT  JP1E  [JP1]
C41  0.1uF  C-EUC0603  [C0603]
C51  4.7uF  C-EUC0603  [C0603]
C52  0.1uF  C-EUC0603  [C0603]
C54  0.1uF  C-EUC0603  [C0603]
C55  10uF  CPOL-USCT3216  [CT3216]
C56  10uF  CPOL-USCT3216  [CT3216]
C57  0.1uF  C-EUC0603  [C0603]
C58  10uF  CPOL-USCT3216  [CT3216]
C59  0.1uF  C-EUC0603  [C0603]
D24  LL103A  D-SOD-80  [SOD80]
D25  LL103A  D-SOD-80  [SOD80]
D26  LL103A  D-SOD-80  [SOD80]
D27  LL103A  D-SOD-80  [SOD80]
EZ-RF  SL127L6TH  [SL127L6_MPE]
IC1  24C02CSN  [SO-08]
IRDA  TFBS4711-TT1  [TFBS4711]
JP11  JP1E  [JP1]
JP12  JP1E  [JP1]
OPTO1  TIL191  [DIL04]
OPTO2  TIL191  [DIL04]
Q1  BC857BSMD  [SOT23-BEC]
Q2  BC857BSMD  [SOT23-BEC]
R47  47  R-EU_R0603  [R0603]
R62  1k  R-EU_R0603  [R0603]
R63  10k  R-EU_R0603  [R0603]
R64  220  R-EU_R0603  [R0603]
R65  68  R-EU_R0603  [R0603]
R66  DNP  R-EU_R0603  [R0603]
R67  1.5k  R-EU_R0603  [R0603]
R68  1k  R-EU_R0603  [R0603]
R69  2.2k  R-EU_R0603  [R0603]
R70  DNP  R-EU_R0603  [R0603]
R71  2.2k  R-EU_R0603  [R0603]
R72  1k  R-EU_R0603  [R0603]
R73  0  R-EU_R0603  [R0603]
R74  0  R-EU_R0603  [R0603]
R75  0  R-EU_R0603  [R0603]
R76  0  R-EU_R0603  [R0603]
R77  0  R-EU_R0603  [R0603]
R78  1k  R-EU_R0603  [R0603]
R79  0  R-EU_R0603  [R0603]
R80  0  R-EU_R0603  [R0603]
R81  0  R-EU_R0603  [R0603]
R82  0  R-EU_R0603  [R0603]
R83  0  R-EU_R0603  [R0603]
R84  0  R-EU_R0603  [R0603]
R85  0  R-EU_R0603  [R0603]
R86  0  R-EU_R0603  [R0603]
R87  0  R-EU_R0603  [R0603]
R88  0  R-EU_R0603  [R0603]
R89  0  R-EU_R0603  [R0603]
R90  0  R-EU_R0603  [R0603]
R91  0  R-EU_R0603  [R0603]
REACT  JP1E  [JP1]
RF1  TFM-110-02-SM-D-A-K  [TFM-110-02-SM-D-A-K]
RF2  TFM-110-02-SM-D-A-K  [TFM-110-02-SM-D-A-K]
RS-232  F09VP  [F09VP]
RX_EN  JP1E  [JP1]
TX_EN  JP1E  [JP1]
U1  PS8802  [SO08]
U2  PS8802  [SO08]

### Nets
ACT: JP12.1 R72.1 ; also sheet 1
DB9_+12V: C54.2 C55.+ D25.1(C) D26.1(C) Q1.E R63.2 U1.8(VCC)
DB9_-12V: C54.1 C56.- D24.2(A) R66.2 R67.1 U1.5(GND)
DB9_GND: C55.- C56.+ D27.2(A) RS-232.5 RS-232.G1 RS-232.G2 U2.3(C)
DGND: C41.1 C51.2 C52.2 C57.2 C58.- C59.1 EZ-RF.5 IC1.1(A0) IC1.2(A1) IC1.3(A2) IC1.4(GND) IC1.7(WP) IRDA.P$6(GND) JP11.2 JP12.2 Q2.C R73.2 R77.2 RF1.2 RF2.1 RF2.19 U2.5(GND) ; also sheet 1,3
DVCC: C41.2 C51.1 C57.1 C58.+ C59.2 EZ-RF.2 IC1.8(VCC) IRDA.P$1(VCC2) OPTO1.1(A) OPTO2.1(A) R47.1 R65.1 R70.2 R71.1 R79.1 RF1.9 U2.8(VCC) ; supply symbol labelled VCC ; also sheet 1,3
EZ-RF_RXD: EZ-RF.6 ; also sheet 1
EZ-RF_TXD: EZ-RF.1 ; also sheet 1
IR_RXD: IRDA.P$3(RXD) ; also sheet 1
IR_SD: IRDA.P$4(SD) ; also sheet 1
IR_TXD: IRDA.P$2(TXD) ; also sheet 1
N$3: ACT.2 OPTO2.4(COL)
N$9: R65.2 U1.2(A)
N$11: ACT.1 OPTO2.3(EMIT)
N$12: OPTO2.2(C) R72.2
N$22: Q2.B R69.2
N$24: R64.1 R67.2 RS-232.2
N$26: R62.1 U1.6(VO)
N$28: Q1.B R62.2 R63.1
N$35: R74.2 RF2.3
N$41: Q1.C R64.2
N$43: R66.1 U1.7(VB)
N$45: R76.2 RF2.5
N$48: C52.1 IRDA.P$5(VCC1) R47.2
N$50: R79.2 RF1.7
N$51: R73.1 RF1.4
N$52: R87.2 RF1.15
N$53: R77.1 RF1.6
N$55: R83.1 RF2.10
N$56: R84.1 RF2.12
N$57: R85.1 RF2.14
N$58: D27.1(C) R78.1 U2.2(A)
N$59: R86.1 RF2.16
N$60: R88.1 RF2.18
N$61: R91.1 RF2.20
N$65: OPTO1.4(COL) REACT.2
N$67: D24.1(C) R78.2 RS-232.3
N$68: OPTO1.3(EMIT) REACT.1
N$69: D26.2(A) RS-232.7
N$71: D25.2(A) RS-232.4
N$72: OPTO1.2(C) R68.2
N$79: Q2.E U1.3(C)
N$81: R90.2 RF1.19
N$83: R89.1 RF1.18
N$85: R80.2 RF2.7
N$86: R82.2 RF2.9
N$87: R81.1 RF2.8
N$88: R75.1 RF2.6
REACT: JP11.1 R68.1 ; also sheet 1
RF_CCA: R83.2 ; also sheet 1
RF_CLK: R86.2 ; also sheet 1
RF_CS: R85.2 ; also sheet 1
RF_FIFO: R75.2 R80.1 ; also sheet 1
RF_FIFOP: R81.2 R82.1 ; also sheet 1
RF_GPIO1: R90.1 ; also sheet 1
RF_GPIO2: R89.2 ; also sheet 1
RF_RESETCC: R76.1 R87.1 ; also sheet 1
RF_SFD: R84.2 ; also sheet 1
RF_SIMO: R88.2 ; also sheet 1
RF_SOMI: R91.2 ; also sheet 1
RF_VREG_EN: R74.1 ; also sheet 1
RS232_RXD: RX_EN.2 ; also sheet 1
RS232_TXD: TX_EN.2 ; also sheet 1
SCL: IC1.6(SCL) ; also sheet 1
SDA: IC1.5(SDA) ; also sheet 1
UART_RX: R70.1 R71.2 RX_EN.1 U2.6(VO)
UART_TX: R69.1 TX_EN.1
Unconnected: EZ-RF.3 EZ-RF.4 RF1.1 RF1.3 RF1.5 RF1.8 RF1.10 RF1.11 RF1.12 RF1.13 RF1.14 RF1.16 RF1.17 RF1.20 RF2.2 RF2.4 RF2.11 RF2.13 RF2.15 RF2.17 RS-232.1 RS-232.6 RS-232.8 RS-232.9 U2.7(VB)

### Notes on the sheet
- Isolated RS232 Communication | IR Pulse In/Out | Act / React
- EEPROM
- EZ-RF Connect
- RF Daughter Card
- TIDM-3PHMTR-TAMP-ESD

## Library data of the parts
ACT JP2 JP11 JP12 REACT RX_EN TX_EN = custom_jumper:JP1E: JUMPER
AUXVCC3 = jumper:JP2E: JUMPER
BTN1-BTN4 RESET = electricalmeter:PB: OMRON SWITCH
C1-C21 C41 C45 C47 C51 C52 C54 C57 C62 = rcl:C-EU: CAPACITOR, European symbol
C22-C38 C40 C42-C44 C48 C49 C53 C59-C61 = resistor:C-EU: CAPACITOR, European symbol
C39 C46 C50 = capacitor-wima:C: CAPACITOR
C55 C56 = resistor:CPOL-US: POLARIZED CAPACITOR, American symbol
C58 C100 = rcl:CPOL-US: POLARIZED CAPACITOR, American symbol
C101 = rcl:CPOL-EU: POLARIZED CAPACITOR, European symbol
C102 = resistor:CPOL-EU: POLARIZED CAPACITOR, European symbol
D1-D16 D28-D44 = FE449x EVM:PMLL4148: DIODE
D17 D19 D21 = diode:1N4757A
D18 D20 D22 = diode:1N4007
D23 = diode:ZENER-DIODE: Z-Diode
D24-D27 = semicon-smd-ipc:D-: DIODE
DGND DVCC = custom_con-lstb:MA04-1: PIN HEADER; OC_FARNELL: unknown; OC_NEWARK: unknown
EZ-RF = susbfet:SL127L6TH
HD1 = SparkFun:M02: Header 2
I1+ I1- I2+ I2- I3+ I3- IN+ IN- LINE1-LINE3 NEUTRAL = testpad:TP: Test pad
IC1 = microchip:24C*: Serial EEPROM 1 K/2 K/4 K; MF: MICROCHIP; MPN: 24C02C/SN; OC_FARNELL: 1607552; OC_NEWARK: 96K4065
IRDA = Personal:TFBS4711-TT1
JP3-JP10 = custom_jumper:JP2E: JUMPER
JP13 = pinhead:PINHD-1X1: PIN HEADER
JTAG = con-ml:ML14: HARTING; OC_FARNELL: unknown; OC_NEWARK: unknown
L1 L3 L5 L6 = FE449x EVM:EXCELSA39: INDUCTOR
L7 = rcl:L-US: INDUCTOR, American symbol
LCD1 = Personal:TI_160SEG_LCD
LED1-LED6 LED_ACT LED_REACT = led:LED: LED
MSP430F67791A = Personal:MSP430F6779IPEU: MSP430F6779IPEU
OPTO1 OPTO2 = optocoupler:TIL191: TEXAS INSTRUMENTS OPTO COUPLER; OC_FARNELL: 1683363; OC_NEWARK: unknown
Q1 Q2 = transistor-pnp:BC857*: PNP Transistror
R1-R3 = varistor:S20K275: VARISTOR
R4-R19 R24-R34 R36 R39 R99-R103 = _MSP430:RES
R20-R23 R35 R37 R38 R92-R95 = resistor:R-US_: RESISTOR, American symbol
R40 R41 R47 R62-R91 = rcl:R-EU_: RESISTOR, European symbol
R42-R46 R48-R61 = resistor:R-EU_: RESISTOR, European symbol
R96-R98 R/L7-R/L14 = rcl:R-US_: RESISTOR, American symbol
RF1 RF2 = _MSP430:TFM-110-02-SM-D-A-K
RS-232 = con-subd:F09VP: SUB-D; OC_FARNELL: unknown; OC_NEWARK: unknown
SV1 = jumper:JP2Q: JUMPER
SV2 = con-lstb:MA05-1: PIN HEADER; OC_FARNELL: unknown; OC_NEWARK: unknown
TVS1-TVS4 = FE449x EVM:SMAJ5.0CA
U1 U2 = FE449x EVM:PS8802: MOTOROLA OPTO COUPLER
U3 = TPS54060:TPS54060_DGQ_10; DATASHEETURL: http://www.ti.com/lit/gpn/TPS54060; DESCRIPTION: 3.5V to 60V Input, 0.5A Step-Down Converter with Eco-Mode; FAMILY_NAME: STEP-DOWN REGULATOR; GENERIC_PART_NUMBER: TPS54060; INDUSTRY_STD_PKG_TYPE: MSOP-PowerPAD; MANUFACTURER: Texas Instruments; MANUFACTURER_PART_NUMBER: tps54060_dgq_10; PACKAGE_DESIGNATOR: DGQ; PIN_COUNT: 10; VENDOR: Texas Instruments
U$1 = TI_MSP430_v16_intern:CUI_XR
XT1 = F20xx PIR Demo & Eval:CM200T
ZD3 = diode:DIODE-: DIODE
